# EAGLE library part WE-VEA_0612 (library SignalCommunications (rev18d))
WE-VEA ESD Suppressor-Array Characteristics Fast response time (1 ns) Low signal insertion loss No leakage current Low clamping voltage Almost no energy consumption in stand-by mode Excellent absorption for ESD-impulses Operating temperature: –40 ºC to +85 ºC Applications Protection of data lines Protection of bus systems Protection of video transmission lines Protection of semiconductors ESD protection in accordance with EN 61000-4-2 Details see: http://katalog.we-online.de/en/pbs/WE-VEA? Updated by Dan Xu 2014-07-11 2014 (C) Wurth Elektronik
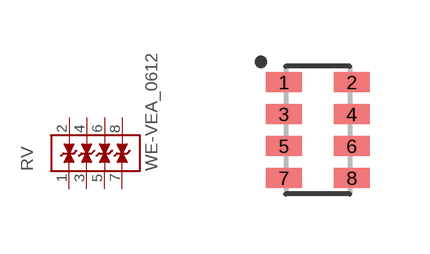
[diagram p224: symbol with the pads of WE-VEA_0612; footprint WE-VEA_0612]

Designator prefix RV

## WE-VEA_0612_82380180121  [WE-VEA_0612]
1  1  pas
2  8  pas
3  2  pas
4  7  pas
5  3  pas
6  6  pas
7  4  pas
8  5  pas

## Footprint WE-VEA_0612 (pad centres in mm)
WESURGE ESD Suppressor-Array WE-VEA
smd 0.9 x 0.5: 1 -0.85,1.2; 2 0.85,1.2; 3 -0.85,0.4; 4 0.85,0.4; 5 -0.85,-0.4; 6 0.85,-0.4; 7 -0.85,-1.2; 8 0.85,-1.2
